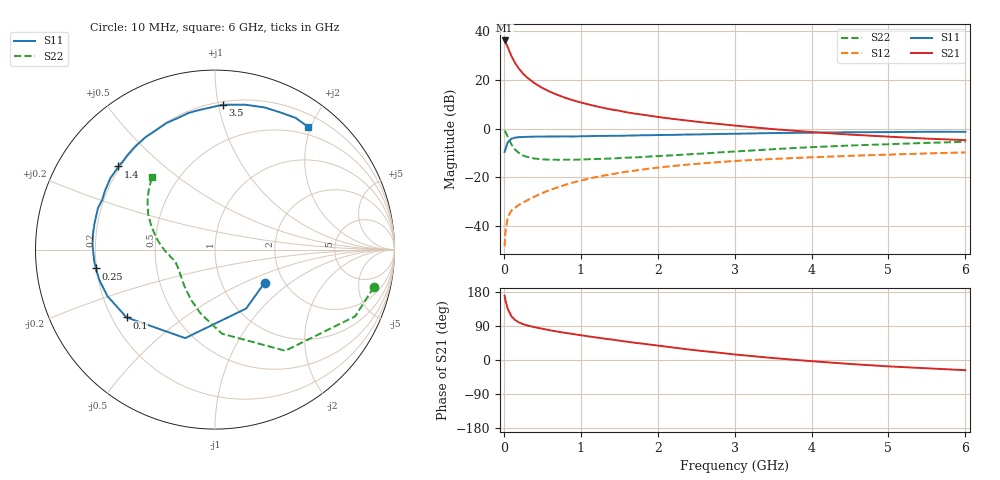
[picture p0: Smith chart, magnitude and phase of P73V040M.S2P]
! SIEMENS Small Signal Semiconductors
! BFP196
! Si NPN RF Bipolar Junction Transistor in SOT143
! VCE = 3 V  IC = 40 mA
! Common Emitter S-Parameters:  May  1996
# GHz  S  MA  R  50
!  f  S11  S21  S12  S22
! GHz  MAG  ANG  MAG  ANG  MAG  ANG  MAG  ANG
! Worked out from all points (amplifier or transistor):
!   36 points, 10 MHz to 6 GHz, reference 50 ohm
!   highest |S21| = 36.1 dB at 10 MHz (marker M1)
!   |S21| within 3 dB of that: start of sweep to 54.72 MHz
!   unconditionally stable (mu >= 1): 485 MHz to 4.048 GHz
!   at 250 MHz: K = 0.80, MSG = 26.4 dB, |S12| = -30.3 dB
!   at 1.4 GHz: K = 1.09, MAG = 11.4 dB, |S12| = -18.7 dB
!   at 6 GHz: K = 0.98, MSG = 2.5 dB, |S12| = -9.8 dB
!   S11 on the Smith chart (normalised r, x): 10 MHz: 1.60, -0.66; 100 MHz: 0.26, -0.32; 250 MHz: 0.20, -0.08; 1.4 GHz: 0.19, +0.36; 3.5 GHz: 0.22, +1.03; 6 GHz: 0.37, +1.95
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0.01  0.3322 -33.6  63.73 169.4  0.0039 80.7  0.909 -13.3
0.02  0.3713 -62.1  59.88 158.3  0.0074 71.4  0.8648 -25.5
0.05  0.5204 -108.6  47.04 135.2  0.0153 57.3  0.6863 -55.2
0.1  0.6208 -142.5  30.26 115.0  0.021 46.7  0.4704 -85.2
0.15  0.653 -156.6  21.48 104.9  0.0242 46.9  0.3655 -102.6
0.2  0.6663 -165.2  16.55 98.9  0.0276 49.0  0.3122 -114.8
0.25  0.6725 -171.0  13.3 94.6  0.0305 51.2  0.2802 -124.3
0.3  0.6766 -175.3  11.18 91.4  0.0337 53.6  0.2632 -130.7
0.4  0.6831 177.7  8.473 86.6  0.0405 56.9  0.2428 -140.8
0.5  0.6852 172.7  6.784 82.5  0.0477 59.1  0.2338 -147.6
0.6  0.6867 168.3  5.664 78.5  0.0555 60.0  0.2304 -152.1
0.7  0.6885 163.8  4.87 74.7  0.0625 60.6  0.2292 -155.6
0.9  0.6867 156.3  3.792 68.5  0.0787 60.0  0.2299 -161.0
1.1  0.6985 149.3  3.12 62.4  0.0938 58.9  0.2351 -164.4
1.4  0.7104 139.3  2.454 54.1  0.1158 55.9  0.2438 -168.6
1.7  0.7219 130.0  2.028 45.5  0.1375 52.1  0.2569 -173.2
2.2  0.742 116.3  1.575 33.0  0.1711 45.0  0.2834 -179.8
2.6  0.7614 105.9  1.33 23.3  0.1949 39.4  0.3089 173.9
3.5  0.8081 87.0  0.974 5.2  0.2386 26.9  0.3774 159.8
4.5  0.8389 70.8  0.752 -10.5  0.2762 15.0  0.449 146.8
5.5  0.8603 58.6  0.622 -21.9  0.3093 4.4  0.5085 135.9
6  0.8585 53.0  0.579 -26.9  0.3247 -1.5  0.5356 130.6
